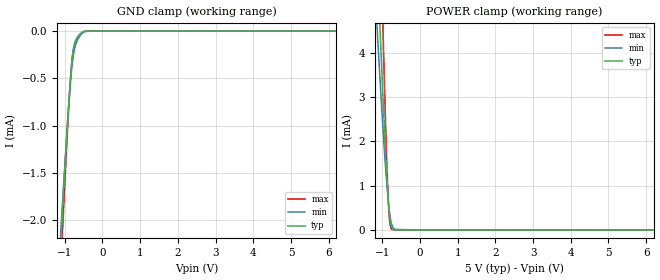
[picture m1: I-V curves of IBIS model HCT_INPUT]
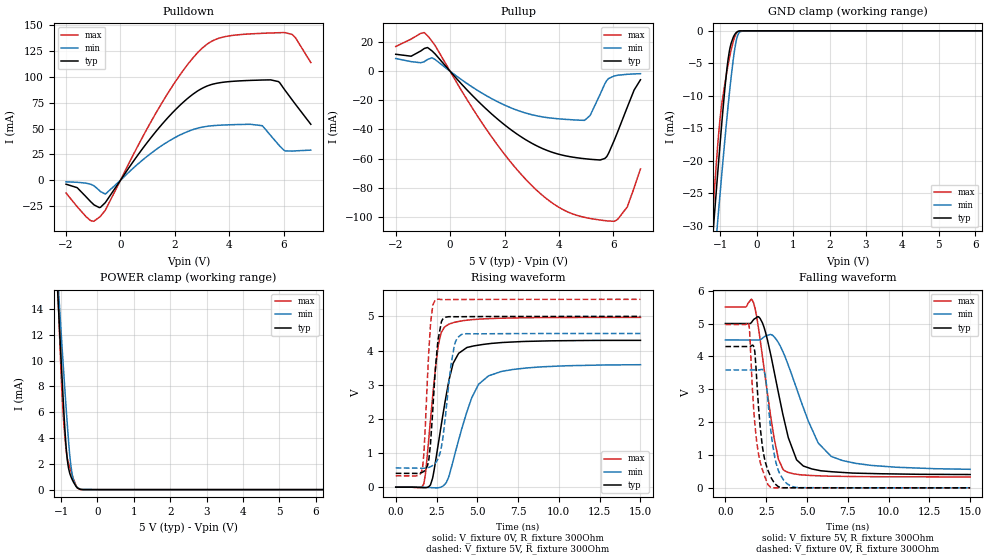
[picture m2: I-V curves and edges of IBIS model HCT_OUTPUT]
| Texas Instruments Incorporated
| SN74HCT240 8-ch, 4.5-V to 5.5-V inverters with TTL-compatible
[IBIS Ver]   4.2
[File name]   sn74hct240.ibs
[Date]   8/2/2022
[File Rev]   0.0
[Source]
[Notes]   Revision History:
[Disclaimer]
| This model is designed as an aid for customers of Texas Instruments.
| TI and its licensors and suppliers make no warranties, either expressed
| or implied, with respect to this  model, including the warranties of
| merchantability or fitness for a particular purpose. The model is
| provided solely on an "as is" basis. The entire risk as to its quality
| and performance is with the customer.
| This model is subject to change without notice. Texas Instruments
| Incorporated is not responsible for updating this model.
[Copyright]
  (C) Copyright 2021 Texas Instruments Incorporated. All rights reserved.
|   Component HCT240_DW
[Component]   HCT240_DW
[Manufacturer]  Texas Instruments, Inc.
[Package]
|   typ   min   max
R_pkg   0.038   0.033   0.045
L_pkg   5.012nH   4.110nH   6.349nH
C_pkg   0.717pF   0.530pF   0.868pF
[Pin]   signal_name   model_name   R_pin   L_pin   C_pin
1   1OE/   input   NA   NA   NA
2   1A1   input   NA   NA   NA
3   2Y4   output   NA   NA   NA
4   1A2   input   NA   NA   NA
5   2Y3   output   NA   NA   NA
6   1A3   input   NA   NA   NA
7   2Y2   output   NA   NA   NA
8   1A4   input   NA   NA   NA
9   2Y1   output   NA   NA   NA
10   GND   GND   NA   NA   NA
11   2A1   input   NA   NA   NA
12   1Y4   output   NA   NA   NA
13   2A2   input   NA   NA   NA
14   1Y3   output   NA   NA   NA
15   2A3   input   NA   NA   NA
16   1Y2   output   NA   NA   NA
17   2A4   input   NA   NA   NA
18   1Y1   output   NA   NA   NA
19   2OE/   input   NA   NA   NA
20   VCC   POWER   NA   NA   NA
| Component HCT240_N 20-pin PDIP
[Component]   HCT240_N
[Manufacturer]   Texas Instruments, Inc.
[Package]
|   typ   min   max
R_pkg   4.300e-02   3.800e-02   5.000e-02
L_pkg   7.384e-09   4.680e-09   1.032e-08
C_pkg   5.100e-13   2.310e-13   8.210e-13
[Pin]   signal_name   model_name   R_pin   L_pin   C_pin
1   1OE/   input   NA   NA   NA
2   1A1   input   NA   NA   NA
3   2Y4   output   NA   NA   NA
4   1A2   input   NA   NA   NA
5   2Y3   output   NA   NA   NA
6   1A3   input   NA   NA   NA
7   2Y2   output   NA   NA   NA
8   1A4   input   NA   NA   NA
9   2Y1   output   NA   NA   NA
10   GND   GND   NA   NA   NA
11   2A1   input   NA   NA   NA
12   1Y4   output   NA   NA   NA
13   2A2   input   NA   NA   NA
14   1Y3   output   NA   NA   NA
15   2A3   input   NA   NA   NA
16   1Y2   output   NA   NA   NA
17   2A4   input   NA   NA   NA
18   1Y1   output   NA   NA   NA
19   2OE/   input   NA   NA   NA
20   VCC   POWER   NA   NA   NA
|   Component HCT240_NS
[Component]   HCT240_NS
[Manufacturer]  Texas Instruments, Inc.
[Package]
|   typ   min   max
R_pkg   0.044   0.029   0.058
L_pkg   3.666nH   2.317nH   5.115nH
C_pkg   0.548pF   0.316pF   0.725pF
[Pin]   signal_name   model_name   R_pin   L_pin   C_pin
1   1OE/   input   NA   NA   NA
2   1A1   input   NA   NA   NA
3   2Y4   output   NA   NA   NA
4   1A2   input   NA   NA   NA
5   2Y3   output   NA   NA   NA
6   1A3   input   NA   NA   NA
7   2Y2   output   NA   NA   NA
8   1A4   input   NA   NA   NA
9   2Y1   output   NA   NA   NA
10   GND   GND   NA   NA   NA
11   2A1   input   NA   NA   NA
12   1Y4   output   NA   NA   NA
13   2A2   input   NA   NA   NA
14   1Y3   output   NA   NA   NA
15   2A3   input   NA   NA   NA
16   1Y2   output   NA   NA   NA
17   2A4   input   NA   NA   NA
18   1Y1   output   NA   NA   NA
19   2OE/   input   NA   NA   NA
20   VCC   POWER   NA   NA   NA
|   Component HCT240_PW
[Component]   HCT240_PW
[Manufacturer]  Texas Instruments, Inc.
[Package]
|   typ   min   max
R_pkg   0.035   0.024   0.047
L_pkg   2.399nH   1.710nH   3.250nH
C_pkg   0.284pF   0.166pF   0.418pF
[Pin]   signal_name   model_name   R_pin   L_pin   C_pin
1   1OE/   input   NA   NA   NA
2   1A1   input   NA   NA   NA
3   2Y4   output   NA   NA   NA
4   1A2   input   NA   NA   NA
5   2Y3   output   NA   NA   NA
6   1A3   input   NA   NA   NA
7   2Y2   output   NA   NA   NA
8   1A4   input   NA   NA   NA
9   2Y1   output   NA   NA   NA
10   GND   GND   NA   NA   NA
11   2A1   input   NA   NA   NA
12   1Y4   output   NA   NA   NA
13   2A2   input   NA   NA   NA
14   1Y3   output   NA   NA   NA
15   2A3   input   NA   NA   NA
16   1Y2   output   NA   NA   NA
17   2A4   input   NA   NA   NA
18   1Y1   output   NA   NA   NA
19   2OE/   input   NA   NA   NA
20   VCC   POWER   NA   NA   NA
|   Model Selectors
[Model Selector] input
HCT_INPUT   5V   digital input
[Model Selector] output
HCT_OUTPUT   5V   digital output
| Models and submodels in the file (2): HCT_INPUT (Input), HCT_OUTPUT (3-state)
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|   HCT_INPUT Model
[Model]   HCT_INPUT
Model_type   Input
Vinl = 0.8
Vinh = 2
|   typ   min   max
C_comp   0.88pF   0.845pF   0.923pF
[Voltage Range]   5   4.5   5.5
[Temperature Range]   27   125   -40
[Power Clamp Reference]   5   4.5   5.5
[GND Clamp Reference]   0   0   0
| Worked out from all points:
|   GND clamp passes 1 mA (typ) near -0.93 V on its own axis
|   POWER clamp passes 1 mA (typ) near -0.86 V on its own axis
[GND Clamp]
|   Voltage   I(typ)   I(min)   I(max)
-2.5V     -13.85mA   -12.44mA   -15.08mA
-1.125V   -2.435mA   -2.249mA   -2.674mA
-1.04V    -1.794mA   -1.682mA   -1.964mA
-935.5mV  -1.039mA   -1.02mA    -1.119mA
-883mV    -698.5uA   -723.6uA   -734.6uA
-830.5mV  -408.5uA   -468.9uA   -412.6uA
-788.5mV  -238.6uA   -310.1uA   -242.9uA
-746.5mV  -139.5uA   -200.4uA   -162.5uA
-694mV    -82.61uA   -121.1uA   -113.4uA
-526mV    -9.336uA   -18.28uA   -14.22uA
-22mV     0A         0A         0A
8V        0A         0A         0A
[POWER Clamp]
|   Voltage   I(typ)   I(min)   I(max)
-2.5V     44.53mA    31.12mA    80.34mA
-1.292V   9.37mA     6.994mA    15.52mA
-1.093V   5.211mA    3.894mA    8.385mA
-1.072V   4.786mA    3.582mA    7.654mA
-1.009V   3.541mA    2.673mA    5.503mA
-946mV    2.357mA    1.826mA    3.452mA
-893.5mV  1.455mA    1.195mA    1.898mA
-841mV    699.4uA    671.1uA    670uA
-799mV    279.6uA    355uA      157uA
-746.5mV  50.25uA    115.3uA    14.45uA
-22mV     0A         0A         0A
8V        0A         0A         0A
[Model]   HCT_OUTPUT
Model_type   3-state
Polarity   Non-Inverting
Vmeas = 2.5
Vref = 2.5
Cref = 15pF
Rref = 100000
|   typ   min   max
C_comp   1.82pF   1.82pF   1.82pF
[Voltage Range]   5   4.5   5.5
[Temperature Range]   25   125   -55
[Pullup Reference]   5   4.5   5.5
[Pulldown Reference]   0   0   0
[Power Clamp Reference]   5   4.5   5.5
[GND Clamp Reference]   0   0   0
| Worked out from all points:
|   slope of the pulldown table from 0 to 0.75 V, typ, clamps not added: 26.4 ohm
|   slope of the pullup table from 0 to 0.75 V, typ, clamps not added: 48.9 ohm
|   GND clamp passes 1 mA (typ) near -0.65 V on its own axis
|   POWER clamp passes 1 mA (typ) near -0.73 V on its own axis
|   falling waveform, V_fixture 5V, R_fixture 300Ohm: 20-80 % time 1.24ns typ, 1.85ns min, 905ps max; typ from 5 V to 0.405 V
|   rising waveform, V_fixture 0V, R_fixture 300Ohm: 20-80 % time 946ps typ, 1.44ns min, 616ps max; typ from 0 V to 4.3 V
|   rising waveform, V_fixture 5V, R_fixture 300Ohm: 20-80 % time 408ps typ, 575ps min, 323ps max; typ from 0.405 V to 5 V
|   falling waveform, V_fixture 0V, R_fixture 300Ohm: 20-80 % time 511ps typ, 557ps min, 485ps max; typ from 4.3 V to 0 V
[Pulldown]
|   Voltage   I(typ)   I(min)   I(max)
-2V       -3.78mA    -1.466mA   -12.32mA
-1.595V   -7.111mA   -1.924mA   -25.45mA
-1.109V   -20.32mA   -3.7mA     -38.82mA
-731mV    -26.07mA   -10.92mA   -34.67mA
-551mV    -21.38mA   -13.27mA   -28.7mA
1.771V    61.41mA    37.82mA    85.42mA
2.662V    83.25mA    49.04mA    118.3mA
3.355V    92.76mA    52.76mA    134.6mA
5.218V    97.07mA    52.82mA    142.3mA
5.812V    95.54mA    34.51mA    142.9mA
6.325V    77.46mA    28.32mA    141mA
7V        54.22mA    29.21mA    114mA
[GND Clamp]
|   Voltage   I(typ)   I(min)   I(max)
-2V       -91.2mA    -92.25mA   -96.76mA
-1.235V   -33.44mA   -39.89mA   -30.11mA
-1.199V   -30.81mA   -37.48mA   -27.16mA
-1.163V   -28.2mA    -35.09mA   -24.27mA
-1.082V   -22.4mA    -29.75mA   -18.11mA
-974mV    -14.96mA   -22.77mA   -11.73mA
-875mV    -8.719mA   -16.59mA   -8.06mA
-785mV    -4.215mA   -11.32mA   -5.108mA
-641mV    -916.3uA   -4.14mA    -1.545mA
-533mV    -132uA     -832.6uA   -171.2uA
-353mV    -379.7nA   -7.593uA   -41.75nA
7V        0A         0A         0A
[Pullup]
|   Voltage   I(typ)   I(min)   I(max)
-2V       11.7mA     8.788mA    17.02mA
-1.433V   10.36mA    6.631mA    22.14mA
-947mV    15.69mA    6.635mA    26.49mA
-668mV    14.02mA    9.263mA    20.72mA
1.141V    -22.63mA   -14.66mA   -34.57mA
2.491V    -43.55mA   -26.94mA   -68.25mA
3.769V    -55.76mA   -32.28mA   -90.68mA
4.948V    -60.09mA   -33.69mA   -100.4mA
5.686V    -59.95mA   -8.746mA   -102.6mA
6.127V    -43.21mA   -2.847mA   -102.2mA
6.514V    -24.74mA   -2.063mA   -93.25mA
7V        -5.831mA   -1.663mA   -67.11mA
[POWER Clamp]
|   Voltage   I(typ)   I(min)   I(max)
-2V       68.05mA    58.49mA    93.08mA
-1.208V   21.72mA    21.72mA    24.9mA
-1.055V   13.13mA    14.68mA    12.96mA
-1.019V   11.14mA    13.06mA    10.26mA
-956mV    7.723mA    10.28mA    6.475mA
-893mV    4.539mA    7.595mA    3.965mA
-830mV    2.339mA    5.068mA    2.441mA
-767mV    1.316mA    2.823mA    1.777mA
-695mV    780.7uA    1.169mA    1.116mA
-659mV    573.6uA    716.9uA    803.3uA
-542mV    110.4uA    137.1uA    97.94uA
7V        0A         0A         0A
[Ramp]
R_load = 300
|   typ   min   max
dV/dt_r   2.57916/9.45786e-10   2.15126/1.43859e-09   2.98267/6.16224e-10
dV/dt_f   2.7568/1.24359e-09   2.36176/1.8451e-09   3.10109/9.04597e-10
[Falling Waveform]
V_fixture = 5V
V_fixture_min = 4.5V
V_fixture_max = 5.5V
R_fixture = 300Ohm
C_fixture = 0F
|   Time   V(typ)   V(min)   V(max)
0s        5V         4.5V       5.5V
1.73ns    5.119V     4.499V     5.624V
2.393ns   4.845V     4.6V       3.545V
2.989ns   3.537V     4.592V     1.504V
3.251ns   2.888V     4.415V     871.5mV
3.624ns   2.02V      4.028V     523.4mV
4.363ns   852.7mV    3.022V     414mV
5.686ns   535.8mV    1.365V     366.8mV
6.485ns   491.3mV    955mV      354.1mV
15ns      405.4mV    563.6mV    331.5mV
[Rising Waveform]
V_fixture = 0V
V_fixture_min = 0V
V_fixture_max = 0V
R_fixture = 300Ohm
C_fixture = 0F
|   Time   V(typ)   V(min)   V(max)
0s        126uV      291.6uV    64.95uV
1.73ns    -16.22mV   -656.3uV   110.5mV
2.129ns   67.68mV    -11.64mV   1.969V
2.607ns   1.263V     -16.12mV   4.156V
2.989ns   2.401V     76.14mV    4.689V
3.517ns   3.625V     771.3mV    4.815V
3.856ns   3.919V     1.381V     4.853V
4.659ns   4.123V     2.619V     4.904V
5.686ns   4.199V     3.259V     4.934V
15ns      4.299V     3.586V     4.971V
[Rising Waveform]
V_fixture = 5V
V_fixture_min = 4.5V
V_fixture_max = 5.5V
R_fixture = 300Ohm
C_fixture = 0F
|   Time   V(typ)   V(min)   V(max)
0s        405.1mV    563.7mV    331.5mV
1.647ns   440.5mV    555.9mV    578.2mV
1.73ns    466mV      555.8mV    1.003V
1.955ns   645.1mV    567.1mV    3.284V
2.136ns   1.309V     599.5mV    4.804V
2.437ns   3.49V      712mV      5.497V
2.801ns   4.848V     1.186V     5.494V
3.595ns   4.991V     4.156V     5.494V
4.042ns   4.991V     4.475V     5.496V
15ns      5V         4.5V       5.5V
[Falling Waveform]
|Gnd
V_fixture = 0V
V_fixture_min = 0V
V_fixture_max = 0V
R_fixture = 300Ohm
C_fixture = 0F
|   Time   V(typ)   V(min)   V(max)
0s        4.299V     3.586V     4.971V
1.439ns   4.298V     3.587V     4.971V
1.753ns   4.276V     3.587V     2.278V
1.92ns    3.291V     3.587V     1.394V
2.129ns   1.859V     3.594V     792.9mV
2.442ns   798.2mV    3.43V      306.7mV
2.78ns    335mV      1.76V      13.89mV
3.229ns   43.11mV    551mV      661.1uV
4.042ns   2.292mV    45.75mV    1.617mV
15ns      130.9uV    291.7uV    64.95uV
